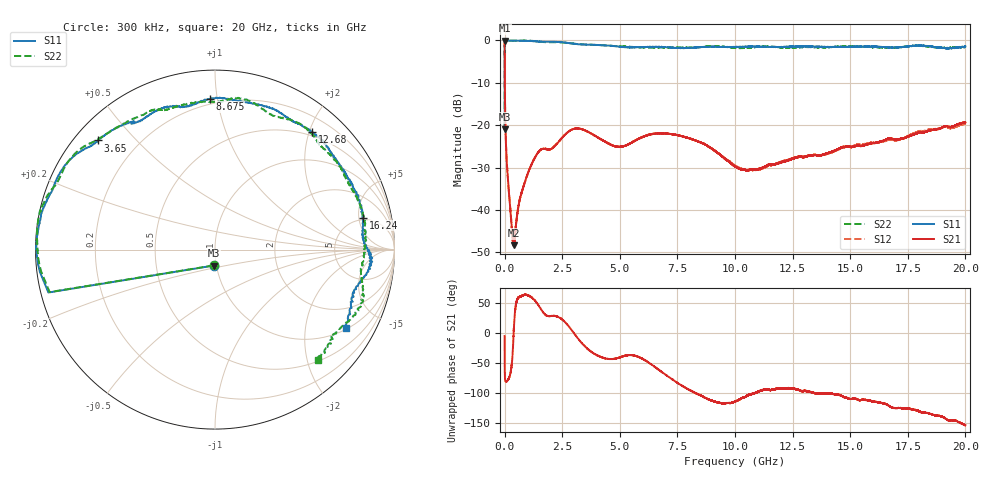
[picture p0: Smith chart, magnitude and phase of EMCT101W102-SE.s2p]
!EMCT101W102
!Johanson Technology Inc.
!www.johansontechnology.com
!Test Board Conditions:
!Substrate Type  RO4350B
!Substrate Thickness  10 mil
!Substrate Dk  3.66
!TL Type: GCPW
!TL Trace Width  22 mil
!TL Gap  14 mil
!PART MODE SINGLE ENDED (AKA BYPASS)
!DUT TOPOLOGY	SERIES-SHUNT
# MHz S  dB  R 50
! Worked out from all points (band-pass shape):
!   20001 points, 300 kHz to 20 GHz, reference 50 ohm
!   highest |S21| = -0.06 dB at 300 kHz (marker M1); lowest = -48.4 dB at 390.3 MHz (marker M2)
!   |S21| within 3 dB of the highest: start of sweep to 3.362 MHz
!   lowest |S11| = -21.0 dB at 300 kHz (marker M3), VSWR 1.20, Z = 48.4 - j8.7 ohm
!   |S11| at or under -10 dB: start of sweep to 1.212 MHz
!   |S22| runs from -21.0 to 0.0 dB; largest |S21 - S12| = 0.0065
!   S11 on the Smith chart (normalised r, x): 300 kHz: 0.97, -0.17; 3.65 GHz: 0.07, +0.39; 8.675 GHz: 0.17, +0.95; 12.68 GHz: 0.43, +2.04; 16.24 GHz: 4.61, +5.68; 20 GHz: 1.06, -3.31
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0.3  -20.97 -95.1  -0.06 -5.2  -0.05 -5.2  -21.02 -95.2
101.298  -0.05 -179.0  -29.34 -80.0  -29.30 -80.2  -0.11 -178.9
139.298  -0.04 180.0  -32.49 -78.4  -32.44 -78.4  -0.09 -179.9
301.295  -0.04 177.5  -43.56 -54.6  -43.49 -54.9  -0.07 177.3
390.294  -0.06 176.5  -48.35 -2.6  -47.97 -2.3  -0.06 176.1
750.289  -0.08 172.3  -35.67 61.5  -35.67 61.7  -0.01 171.0
1404.279  -0.21 163.6  -26.81 49.7  -26.79 50.1  -0.20 161.5
2080.269  -0.31 155.1  -25.39 28.5  -25.34 28.3  -0.41 152.4
2869.257  -0.68 143.5  -21.16 7.0  -21.18 6.7  -0.68 141.2
3334.25  -0.94 139.4  -20.91 -16.1  -20.92 -15.9  -0.90 137.8
3650.245  -1.00 137.0  -21.64 -27.7  -21.64 -27.8  -0.99 136.2
4961.226  -1.43 122.6  -25.09 -41.2  -25.13 -41.1  -1.39 118.4
6667.2  -1.51 109.6  -21.98 -60.4  -21.92 -60.6  -1.66 105.3
8675.17  -1.51 92.0  -24.42 -107.2  -24.47 -107.3  -1.48 84.3
10000.15  -1.53 77.2  -29.73 -113.8  -29.52 -114.1  -1.71 69.2
10964.14  -1.43 66.9  -30.44 -98.3  -30.54 -98.9  -1.55 59.1
12677.11  -1.41 50.6  -27.55 -93.9  -27.55 -94.0  -1.62 39.7
13334.1  -1.46 42.5  -27.07 -98.6  -27.11 -99.1  -1.58 31.4
16240.06  -1.48 12.2  -23.95 -115.1  -24.03 -116.8  -1.60 -1.8
16667.05  -1.65 6.9  -23.16 -120.8  -23.41 -120.6  -1.71 -6.7
17898.03  -1.25 -4.2  -21.90 -128.8  -21.68 -128.0  -1.29 -20.6
20000  -1.42 -30.8  -19.33 -153.4  -19.57 -150.7  -1.56 -46.9
